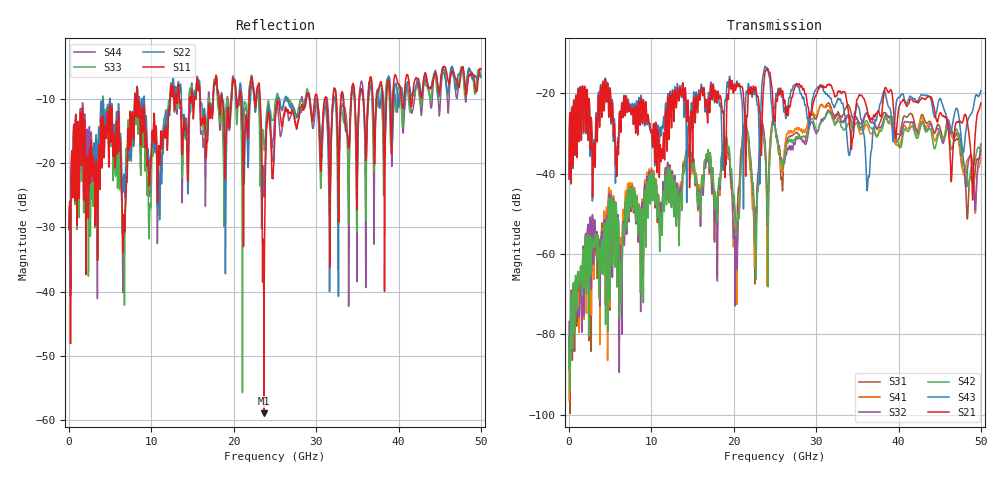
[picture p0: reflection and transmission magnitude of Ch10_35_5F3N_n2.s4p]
!Agilent Technologies,N5247A,US51170199,A.09.90.13
!Agilent N5247A: A.09.90.13
!Date: Tuesday, December 08, 2015 12:07:52
!Correction: S11(Full 4 Port(1,2,3,4))
!S12(Full 4 Port(1,2,3,4))
!S13(Full 4 Port(1,2,3,4))
!S14(Full 4 Port(1,2,3,4))
!S21(Full 4 Port(1,2,3,4))
!S22(Full 4 Port(1,2,3,4))
!S23(Full 4 Port(1,2,3,4))
!S24(Full 4 Port(1,2,3,4))
!S31(Full 4 Port(1,2,3,4))
!S32(Full 4 Port(1,2,3,4))
!S33(Full 4 Port(1,2,3,4))
!S34(Full 4 Port(1,2,3,4))
!S41(Full 4 Port(1,2,3,4))
!S42(Full 4 Port(1,2,3,4))
!S43(Full 4 Port(1,2,3,4))
!S44(Full 4 Port(1,2,3,4))
!S4P File: Measurements: <S11,S12,S13,S14>,
!<S21,S22,S23,S24>,
!<S31,S32,S33,S34>,
!<S41,S42,S43,S44>:
# Hz S  dB  R 50
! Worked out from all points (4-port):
!   3201 points, 10 MHz to 50 GHz, reference 50 ohm
!   strongest paths, dB at 10 MHz, 12.51 GHz, 25 GHz, 37.5 GHz, 50 GHz:
!     S21: -41.2, -21.8, -26.8, -24.3, -22.4
!     S43: -41.4, -21.0, -23.2, -24.7, -19.3
!     S42: -80.9, -40.4, -28.5, -30.4, -32.5
!     S32: -76.8, -39.9, -27.8, -28.6, -32.8
!     S41: -96.5, -39.4, -28.3, -30.3, -35.7
!     S31: -88.0, -40.6, -27.9, -28.6, -34.0
!   lowest |S11| = -58.9 dB at 23.66 GHz (marker M1), VSWR 1.00, Z = 49.9 + j0.0731 ohm
!   |S11| at or under -10 dB: start of sweep to 7.975 GHz; 8.343 GHz to 12.29 GHz (3.946 GHz wide, 38.3 % of centre); 23.2 GHz to 28.8 GHz (5.593 GHz wide, 21.5 % of centre)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
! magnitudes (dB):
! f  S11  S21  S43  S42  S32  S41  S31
! 10 MHz  -30.2  -41.2  -41.4  -80.9  -76.8  -96.5  -88.0
! 7.54 GHz  -17.4  -24.9  -25.2  -48.0  -48.9  -46.3  -49.4
! 22.19 GHz  -6.6  -19.8  -20.7  -40.7  -40.6  -44.6  -42.8
! 23.66 GHz  -58.9  -17.5  -14.5  -31.1  -29.5  -31.5  -30.5
! 36.3 GHz  -10.5  -25.2  -41.5  -27.4  -25.7  -28.4  -25.5
! 38.21 GHz  -15.7  -20.5  -19.4  -27.4  -26.5  -26.8  -24.8
! 50 GHz  -5.4  -22.4  -19.3  -32.5  -32.8  -35.7  -34.0
